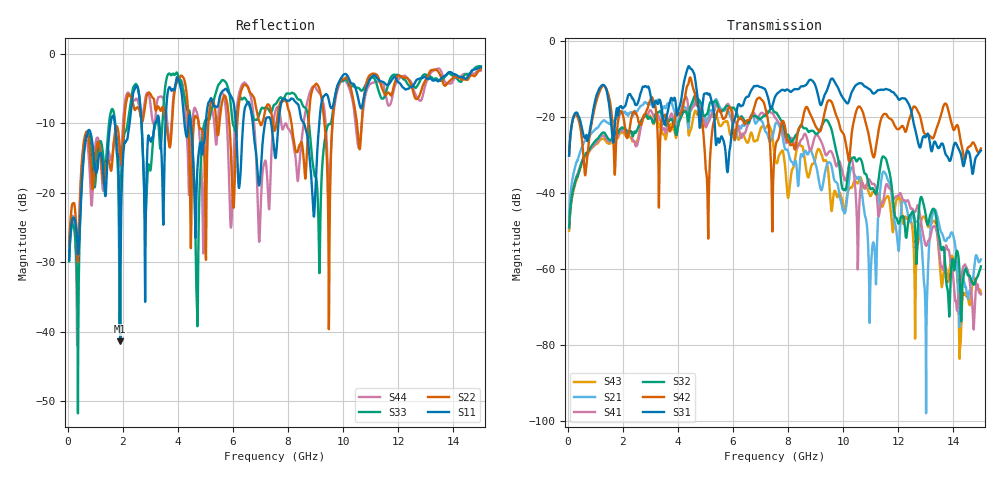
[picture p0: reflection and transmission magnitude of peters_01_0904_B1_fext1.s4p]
# MHZ S RI R 50.00
! FREQ  S11  S12  S13  S14
!  S21  S22  S23  S24
!  S31  S32  S33  S34
!  S41  S42  S43  S44
!  REAL  IMAG  REAL  IMAG  REAL  IMAG  REAL  IMAG
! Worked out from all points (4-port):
!   1496 points, 50 MHz to 15 GHz, reference 50 ohm
!   strongest paths, dB at 50 MHz, 3.79 GHz, 7.53 GHz, 11.27 GHz, 15 GHz:
!     S31: -30.1, -15.2, -14.6, -12.8, -28.8
!     S42: -29.9, -22.5, -28.4, -24.1, -28.2
!     S32: -49.0, -20.6, -18.7, -37.2, -59.2
!     S41: -49.1, -19.2, -20.1, -45.3, -66.6
!     S21: -45.7, -16.5, -22.0, -45.9, -57.4
!     S43: -49.8, -22.2, -31.2, -40.0, -66.1
!   lowest |S11| = -41.4 dB at 1.91 GHz (marker M1), VSWR 1.02, Z = 50.5 - j0.711 ohm
!   |S11| at or under -10 dB: start of sweep to 1.554 GHz; 4.468 GHz to 5.013 GHz (544.3 MHz wide, 11.5 % of centre); 8.577 GHz to 9.132 GHz (555.5 MHz wide, 6.27 % of centre)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
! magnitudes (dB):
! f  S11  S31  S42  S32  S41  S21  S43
! 50 MHz  -29.7  -30.1  -29.9  -49.0  -49.1  -45.7  -49.8
! 1.91 GHz  -41.4  -17.2  -18.5  -23.1  -23.6  -19.1  -24.2
! 9.4 GHz  -5.8  -13.1  -16.6  -20.7  -30.0  -32.6  -31.7
! 10.98 GHz  -3.6  -12.7  -26.9  -38.8  -36.7  -65.7  -40.7
! 11.48 GHz  -4.1  -12.7  -19.1  -30.4  -41.0  -34.3  -42.3
! 12.99 GHz  -3.4  -25.2  -24.5  -45.3  -53.6  -72.4  -46.7
! 15 GHz  -1.9  -28.8  -28.2  -59.2  -66.6  -57.4  -66.1
